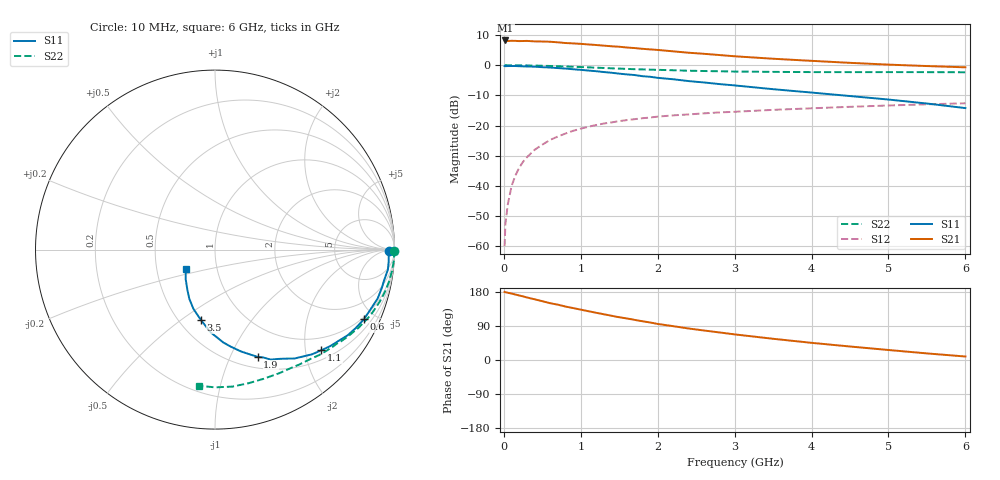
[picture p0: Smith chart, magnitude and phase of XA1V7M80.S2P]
! SIEMENS Discrete & RF Semiconductors
! BFY180
! Si NPN RF Bipolar Junction Transistor in MICRO-X
! VCE = 1.75 V  IC = 0.8 mA
! Common Emitter S-Parameters:  May  1997
# GHz  S  MA  R  50
!  f  S11  S21  S12  S22
! GHz  MAG  ANG  MAG  ANG  MAG  ANG  MAG  ANG
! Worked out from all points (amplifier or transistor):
!   36 points, 10 MHz to 6 GHz, reference 50 ohm
!   highest |S21| = 8.2 dB at 20 MHz (marker M1)
!   |S21| within 3 dB of that: start of sweep to 1.923 GHz
!   unconditionally stable (mu >= 1): 3.913 GHz to end of sweep
!   at 250 MHz: K = 0.08, MSG = 20.0 dB, |S12| = -32.0 dB
!   at 1.4 GHz: K = 0.49, MSG = 12.6 dB, |S12| = -19.0 dB
!   at 6 GHz: K = 1.07, MAG = 4.4 dB, |S12| = -12.6 dB
!   S11 on the Smith chart (normalised r, x): 10 MHz: 61, -10; 600 MHz: 0.90, -4.35; 1.1 GHz: 0.70, -2.34; 1.9 GHz: 0.62, -1.27; 3.5 GHz: 0.64, -0.60; 6 GHz: 0.71, -0.16
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0.01  0.9684 -0.3  2.532 179.7  0.001 93.0  0.9974 -0.3
0.02  0.963 -1.0  2.574 178.9  0.0023 94.1  0.9999 -0.5
0.05  0.9686 -2.1  2.521 177.6  0.0048 87.5  0.9981 -1.3
0.1  0.9699 -4.2  2.542 175.3  0.0099 87.5  0.998 -2.6
0.15  0.9698 -6.6  2.533 172.8  0.0148 85.7  0.9976 -3.9
0.2  0.964 -8.2  2.511 170.2  0.02 83.9  0.9956 -5.1
0.3  0.9541 -12.7  2.53 165.0  0.0298 80.9  0.9912 -7.7
0.4  0.9465 -16.7  2.485 160.2  0.0396 77.8  0.9864 -10.2
0.6  0.9168 -24.9  2.452 149.9  0.0576 72.1  0.9718 -15.1
0.9  0.8575 -36.2  2.3 137.1  0.0817 63.6  0.9434 -22.1
1.1  0.816 -43.4  2.209 128.7  0.0955 58.8  0.9211 -26.3
1.5  0.725 -56.9  2.025 112.8  0.1183 50.1  0.8788 -34.1
1.9  0.6433 -68.3  1.831 99.1  0.1358 43.4  0.8443 -40.8
2  0.6176 -71.3  1.793 95.2  0.1405 41.9  0.8385 -42.3
2.2  0.5856 -75.7  1.7 89.3  0.1474 39.0  0.8253 -45.5
2.4  0.5462 -81.0  1.612 83.2  0.1528 36.5  0.811 -48.3
2.8  0.4871 -89.0  1.476 72.8  0.1649 32.2  0.7939 -53.8
3.5  0.4005 -101.2  1.281 56.0  0.182 25.7  0.7757 -62.8
4  0.3521 -109.9  1.182 45.3  0.1931 21.4  0.7691 -69.3
4.5  0.3085 -117.7  1.095 35.6  0.2044 17.3  0.7676 -76.0
5.5  0.2317 -134.8  0.969 17.4  0.2249 9.3  0.7675 -89.9
6  0.1947 -146.7  0.923 9.2  0.2339 5.0  0.7643 -96.9
